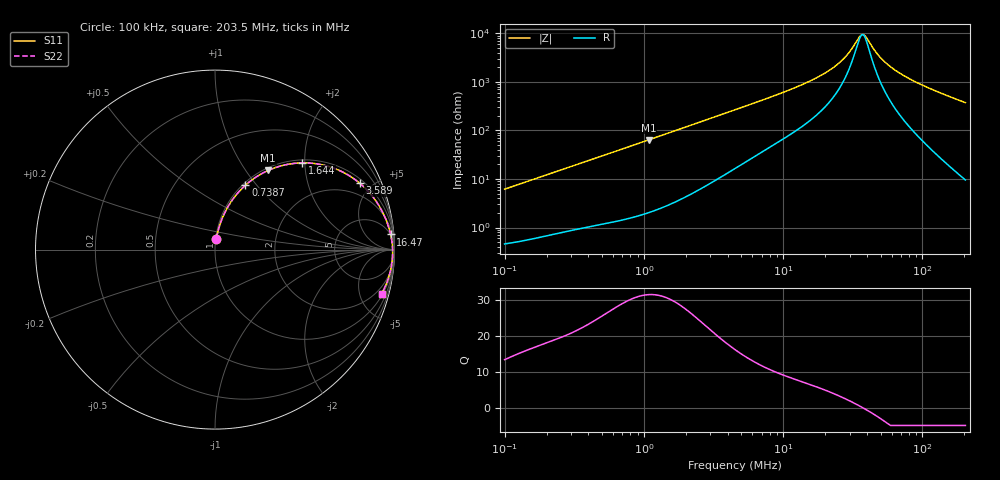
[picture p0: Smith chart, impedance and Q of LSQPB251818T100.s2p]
! LSQPB251818T100  S-PARAMETER MODEL  ( General Type )
! Model Generated by TAIYO YUDEN Corporation (http://www.ty-top.com)
! Version 2.0
! TAIYO YUDEN Control No. 100810NG19SB-FKC
! Copyright(c) 2009 TAIYO YUDEN CO.,LTD. All Rights Reserved.
! Product Description (link to TY-COMPAS)
! https://ds.yuden.co.jp/TYCOMPAS/or/detail?pn=LSQPB251818T100K&u=M
! Products Name : Inductors
! Characteristics :
!  Inductance : 10 uH , SRF(min) : 20 MHz , DC Resistance(max) : 0.455 Ohm
!  Rated Current : Saturation :890 mA , Temp Rise : 610 mA (40 degC)
!  Case Size : 2.5 x 1.8 / 0.098 x 0.071 [mm/inch] , Thickness : 1.8 / 0.071 [mm/inch]
!  (Conditions: Temperature = 25 degC , DC Bias Current/Voltage = 0A / 0V)
! External Node Assignments :
!  1  o---GGG---o  2
! GND o---------o GND
! Frequency Range : 0.1MHz  -  203.457813MHz  [ 402 STEP ]
# MHz S RI R 50
! Freq[MHz].  S11 Real  S11 Imag  S21 Real  S21 Imag  S12 Real  S12 Imag  S22 Real  S22 Imag
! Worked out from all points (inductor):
!   401 points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, 100 kHz to 203.5 MHz, reference 50 ohm
!   read as one part in series: L = 9.75 uH near 103.9 kHz
!   highest Q = 31.6 at 1.081 MHz (marker M1), where L = 9.4 uH
!   self-resonance near 36.65 MHz
!   S11 on the Smith chart (normalised r, x): 100 kHz: 1.01, +0.12; 738.7 kHz: 1.03, +0.87; 1.644 MHz: 1.07, +1.94; 3.589 MHz: 1.22, +4.23; 16.47 MHz: 5, +22; 203.5 MHz: 1.19, -7.47
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0.1  0.00829 0.0607  0.9917 -0.0607  0.9917 -0.0607  0.00829 0.0607
0.358236  0.0524 0.2015  0.9476 -0.2015  0.9476 -0.2015  0.0524 0.2015
0.738711  0.169 0.3582  0.831 -0.3582  0.831 -0.3582  0.169 0.3582
1.081181  0.2956 0.4408  0.7044 -0.4408  0.7044 -0.4408  0.2956 0.4408
1.283332  0.3687 0.4668  0.6313 -0.4668  0.6313 -0.4668  0.3687 0.4668
1.643858  0.4851 0.4832  0.5149 -0.4832  0.5149 -0.4832  0.4851 0.4832
2.316038  0.6455 0.4592  0.3545 -0.4592  0.3545 -0.4592  0.6455 0.4592
3.589078  0.8053 0.3707  0.1947 -0.3707  0.1947 -0.3707  0.8053 0.3707
4.51063  0.8618 0.3156  0.1382 -0.3156  0.1382 -0.3156  0.8618 0.3156
9.662391  0.9557 0.159  0.0443 -0.159  0.0443 -0.159  0.9557 0.159
16.15871  0.9781 0.0868  0.0219 -0.0868  0.0219 -0.0868  0.9781 0.0868
16.4694  0.9786 0.0845  0.0214 -0.0845  0.0214 -0.0845  0.9786 0.0845
21.50178  0.9844 0.0545  0.0156 -0.0545  0.0156 -0.0545  0.9844 0.0545
26.01275  0.9871 0.0348  0.0129 -0.0348  0.0129 -0.0348  0.9871 0.0348
29.16174  0.9882 0.0234  0.0118 -0.0234  0.0118 -0.0234  0.9882 0.0234
34.61418  0.9893 0.00676  0.0107 -0.00676  0.0107 -0.00676  0.9893 0.00676
36.64946  0.9896 0.00123  0.0104 -0.00123  0.0104 -0.00123  0.9896 0.00123
38.80442  0.9897 -0.00431  0.0103 0.00431  0.0103 0.00431  0.9897 -0.00431
47.84805  0.9896 -0.025  0.0104 0.025  0.0104 0.025  0.9896 -0.025
57.88634  0.9886 -0.0448  0.0114 0.0448  0.0114 0.0448  0.9886 -0.0448
94.97886  0.9803 -0.1055  0.0197 0.1055  0.0197 0.1055  0.9803 -0.1055
203.4578  0.9278 -0.2464  0.0722 0.2464  0.0722 0.2464  0.9278 -0.2464
